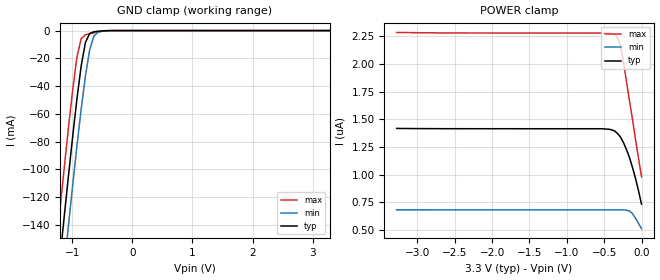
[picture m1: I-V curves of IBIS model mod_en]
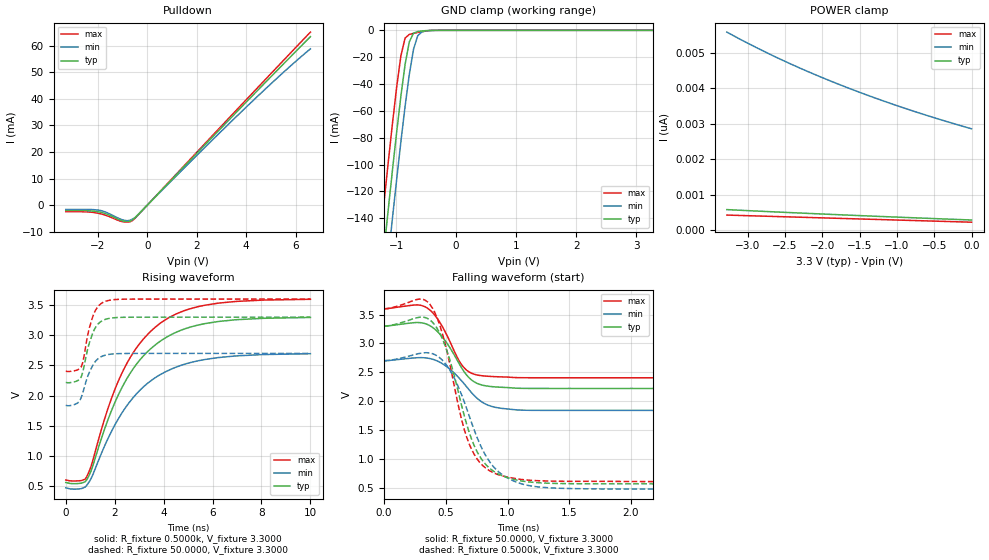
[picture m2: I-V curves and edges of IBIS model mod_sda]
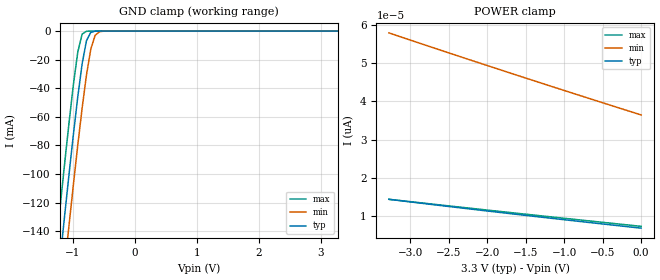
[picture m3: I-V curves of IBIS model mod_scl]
| IBIS (I/O, Buffer, Information, Specification) Model, officially
| electronic behavioral standard for Buffer structures of digital pins.
[IBIS ver]  4.0
[File name] m24c32_fd2_tssop8.ibs
[File Rev]  1.0
[Date]   2 March 2015
[Source]   CAD & Design Services (Catania) - STMicroelectronics
[Notes]
   (Note1)  This IBIS model includes the TSSOP8 Package data
   (Note2)  This IBIS model has some Notes about the non-monotonicity
   of the I-V curves, but they are not indicative of problems
   inside the model;
[Copyright] (c) 2015 STMicroelectronics
|   Component M24C32
[Component] M24C32
[Manufacturer] STMicroelectronics
[Package]
| variable   typ   min   max
R_pkg   0.0   0.0   0.0
L_pkg   0.0H   0.0H   0.0H
C_pkg   0.0F   0.0F   0.0F
[Pin]   signal_name   model_name   R_pin   L_pin   C_pin
1   E1   mod_en   NA   NA   NA
2   E2   mod_en   NA   NA   NA
3   E3   mod_en   NA   NA   NA
4   VSS   GND   NA   NA   NA
5   SDA   mod_sda   NA   NA   NA
6   SCL   mod_scl   NA   NA   NA
7   WC   mod_wc   NA   NA   NA
8   VCC   POWER   NA   NA   NA
[Package Model]  182696_TSSOP8
[Define Package Model]  182696_TSSOP8
[Manufacturer]  STMicroelectronics
[OEM]  STMicroelectronics
[Description]  8 pin TSSOP package
[Number Of Pins]  8
[Pin Numbers]
|Pin Num   Terminal Name
1   | net1
2   | net2
3   | net3
4   | net4_GND
5   | net5
6   | net6
7   | net7
8   | net8_VDD
[Model Data]
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[End Model Data]
[End Package Model]
| Models and submodels in the file (4): mod_en (Input), mod_sda (I/O_open_drain), mod_scl (Input), mod_wc (Input)
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|   Model mod_en
[Model]   mod_en
Model_type Input
Vinl   =   1.000V
Vinh   =   2.300V
C_comp   1.763pF   1.683pF   1.933pF
[Temperature Range]   25.0000   85.0000   -40.0000
[Voltage Range]   3.3000V   2.7000V   3.6000V
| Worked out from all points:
|   GND clamp passes 1 mA (typ) near -0.65 V on its own axis
[GND_clamp]
|Voltage   I(typ)   I(min)   I(max)
-3.3V     -1.113A    -1.147A    -1.081A
-1.27V    -193.3mA   -229.4mA   -158.1mA
-1.2V     -163.1mA   -199.1mA   -127.8mA
-1.13V    -133.2mA   -169.2mA   -98.1mA
-1.06V    -104mA     -139.7mA   -69.27mA
-920mV    -48.97mA   -82.95mA   -18.95mA
-850mV    -25.39mA   -56.55mA   -5.752mA
-780mV    -8.589mA   -32.8mA    -3.057mA
-710mV    -2.164mA   -14.14mA   -2.277mA
-640mV    -888.1uA   -4.039mA   -1.614mA
-500mV    -222.8uA   -481.2uA   -433uA
3.28V     279.1pA    3.222nA    199.4pA
[POWER_clamp]
|Voltage   I(typ)   I(min)   I(max)
-3.28V    1.419uA    683.7nA    2.286uA
-520mV    1.416uA    682.7nA    2.281uA
-400mV    1.406uA    682.7nA    2.278uA
-360mV    1.396uA    682.7nA    2.269uA
-320mV    1.373uA    682.7nA    2.235uA
-280mV    1.339uA    682.7nA    2.163uA
-240mV    1.288uA    682.7nA    2.015uA
-160mV    1.154uA    672.4nA    1.665uA
-120mV    1.064uA    648nA      1.498uA
-80mV     966.4nA    607.3nA    1.318uA
-40mV     855.2nA    560.8nA    1.15uA
0V        735nA      513nA      982.3nA
|   Model mod_sda
[Model]   mod_sda
Model_type I/O_open_drain
Polarity   Inverting
Vinl   =   1.000V
Vinh   =   2.300V
Vmeas  =   1.250V
Cref   =   10pF
Rref   =   1k
Vref   =   3.300V
C_comp   1.845pF   1.762pF   2.024pF
[Temperature Range]   25.0000   85.0000   -40.0000
[Voltage Range]   3.3000V   2.7000V   3.6000V
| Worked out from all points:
|   slope of the pulldown table from 0 to 0.495 V, typ, clamps not added: 102 ohm
|   GND clamp passes 1 mA (typ) near -0.65 V on its own axis
|   rising waveform, R_fixture 0.5000k, V_fixture 3.3000: 20-80 % time 2.08ns typ, 2.16ns min, 2.02ns max; typ from 0.561 V to 3.29 V
|   rising waveform, R_fixture 50.0000, V_fixture 3.3000: 20-80 % time 435ps typ, 476ps min, 412ps max; typ from 2.22 V to 3.3 V
|   falling waveform, R_fixture 50.0000, V_fixture 3.3000: 20-80 % time 193ps typ, 228ps min, 171ps max; typ from 3.3 V to 2.22 V
|   falling waveform, R_fixture 0.5000k, V_fixture 3.3000: 20-80 % time 230ps typ, 265ps min, 207ps max; typ from 3.3 V to 0.561 V
[Pulldown]
|Voltage   I(typ)   I(min)   I(max)
-3.3V     -2.064mA   -1.658mA   -2.43mA
-2.4V     -2.108mA   -1.658mA   -2.579mA
-2V       -2.482mA   -1.86mA    -3.052mA
-1.7V     -3.183mA   -2.587mA   -3.78mA
-1V       -5.94mA    -5.557mA   -6.235mA
-800mV    -6.205mA   -5.866mA   -6.431mA
-600mV    -5.548mA   -5.296mA   -5.811mA
-400mV    -3.913mA   -3.782mA   -3.987mA
2V        19.48mA    18.7mA     19.89mA
4V        38.78mA    36.89mA    39.67mA
5.5V      53.08mA    49.94mA    54.41mA
6.6V      63.45mA    58.86mA    65.17mA
[GND_clamp]
|Voltage   I(typ)   I(min)   I(max)
-3.3V     -1.113A    -1.147A    -1.081A
-1.27V    -193.3mA   -229.4mA   -158.1mA
-1.2V     -163.1mA   -199.1mA   -127.8mA
-1.13V    -133.2mA   -169.2mA   -98.1mA
-1.06V    -104mA     -139.7mA   -69.27mA
-920mV    -48.97mA   -82.95mA   -18.95mA
-850mV    -25.39mA   -56.55mA   -5.752mA
-780mV    -8.589mA   -32.8mA    -3.057mA
-710mV    -2.164mA   -14.14mA   -2.277mA
-640mV    -888.1uA   -4.039mA   -1.614mA
-500mV    -222.8uA   -481.2uA   -433uA
3.28V     279.1pA    3.222nA    199.4pA
[POWER_clamp]
|Voltage   I(typ)   I(min)   I(max)
-3.28V    574.3pA    5.587nA    419.8pA
-2.92V    537.5pA    5.187nA    397.6pA
-2.56V    502.2pA    4.819nA    375.4pA
-2.16V    464.4pA    4.443nA    350.8pA
-1.76V    428pA      4.097nA    326.3pA
-1.36V    392.9pA    3.778nA    301.8pA
-920mV    355.5pA    3.454nA    275pA
-480mV    319.2pA    3.156nA    248.1pA
0V        280.7pA    2.857nA    218.9pA
[Ramp]
| variable   typ   min   max
dV/dt_r   0.6483/0.5008n   0.5164/0.5520n   0.7169/0.5321n
dV/dt_f   0.6483/0.2217n   0.5163/0.2594n   0.7172/0.2235n
R_load = 50.0000
[Rising Waveform]
R_fixture= 0.5000k
V_fixture= 3.3000
V_fixture_min= 2.7000
V_fixture_max= 3.6000
|time   V(typ)   V(min)   V(max)
0s        560.7mV    472.7mV    601.9mV
850ps     601.6mV    510mV      650.6mV
1.03ns    748.2mV    622.8mV    823mV
1.77ns    1.649V     1.326V     1.84V
2.33ns    2.159V     1.734V     2.402V
3.03ns    2.592V     2.089V     2.867V
3.87ns    2.904V     2.35V      3.202V
4.71ns    3.083V     2.501V     3.387V
5.67ns    3.192V     2.598V     3.497V
10ns      3.295V     2.695V     3.596V
[Rising Waveform]
R_fixture= 50.0000
V_fixture= 3.3000
V_fixture_min= 2.7000
V_fixture_max= 3.6000
|time   V(typ)   V(min)   V(max)
0s        2.219V     1.839V     2.405V
420ps     2.237V     1.863V     2.419V
620ps     2.303V     1.957V     2.47V
720ps     2.434V     2.081V     2.599V
940ps     2.839V     2.363V     3.08V
1.12ns    3.052V     2.512V     3.326V
1.34ns    3.194V     2.617V     3.486V
1.66ns    3.269V     2.675V     3.568V
2.54ns    3.299V     2.699V     3.599V
10ns      3.3V       2.7V       3.6V
[Falling Waveform]
R_fixture= 50.0000
V_fixture= 3.3000
V_fixture_min= 2.7000
V_fixture_max= 3.6000
|time   V(typ)   V(min)   V(max)
0s        3.3V       2.7V       3.6V
260ps     3.363V     2.752V     3.669V
350ps     3.331V     2.747V     3.615V
470ps     3.118V     2.652V     3.301V
590ps     2.72V      2.44V      2.769V
650ps     2.505V     2.297V     2.574V
750ps     2.311V     2.056V     2.455V
870ps     2.252V     1.909V     2.427V
1.23ns    2.22V      1.84V      2.405V
10ns      2.219V     1.839V     2.405V
[Falling Waveform]
R_fixture= 0.5000k
V_fixture= 3.3000
V_fixture_min= 2.7000
V_fixture_max= 3.6000
|time   V(typ)   V(min)   V(max)
0s        3.3V       2.7V       3.6V
280ps     3.452V     2.824V     3.768V
370ps     3.411V     2.834V     3.681V
430ps     3.261V     2.784V     3.443V
510ps     2.866V     2.612V     2.86V
630ps     1.907V     2.099V     1.663V
710ps     1.333V     1.619V     1.158V
870ps     809.3mV    904.6mV    773.9mV
1.09ns    624mV      581mV      647.3mV
10ns      560.7mV    472.7mV    601.9mV
|   Model mod_scl
[Model]   mod_scl
Model_type Input
Vinl   =   1.000V
Vinh   =   2.300V
C_comp   1.763pF   1.683pF   1.933pF
[Temperature Range]   25.0000   85.0000   -40.0000
[Voltage Range]   3.3000V   2.7000V   3.6000V
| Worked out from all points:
|   GND clamp passes 1 mA (typ) near -0.71 V on its own axis
[GND_clamp]
|Voltage   I(typ)   I(min)   I(max)
-3.3V     -1.086A    -1.119A    -1.052A
-1.27V    -186.8mA   -222.8mA   -150.3mA
-1.2V     -157.3mA   -193.3mA   -120.7mA
-1.13V    -128.1mA   -164mA     -91.65mA
-1.06V    -99.56mA   -135.2mA   -63.53mA
-920mV    -45.89mA   -79.74mA   -14.62mA
-850mV    -22.95mA   -53.94mA   -2.113mA
-780mV    -6.754mA   -30.77mA   -106.4uA
-710mV    -883.8uA   -12.62mA   -4.426uA
-640mV    -77.7uA    -2.974mA   -182.3nA
-570mV    -6.449uA   -439.9uA   -7.506nA
3.28V     6.813pA    40.1pA     6.666pA
[POWER_clamp]
|Voltage   I(typ)   I(min)   I(max)
-3.28V    14.38pA    57.84pA    14.39pA
-2.52V    12.55pA    52.74pA    12.71pA
-1.72V    10.69pA    47.47pA    10.97pA
0V        6.856pA    36.42pA    7.331pA
